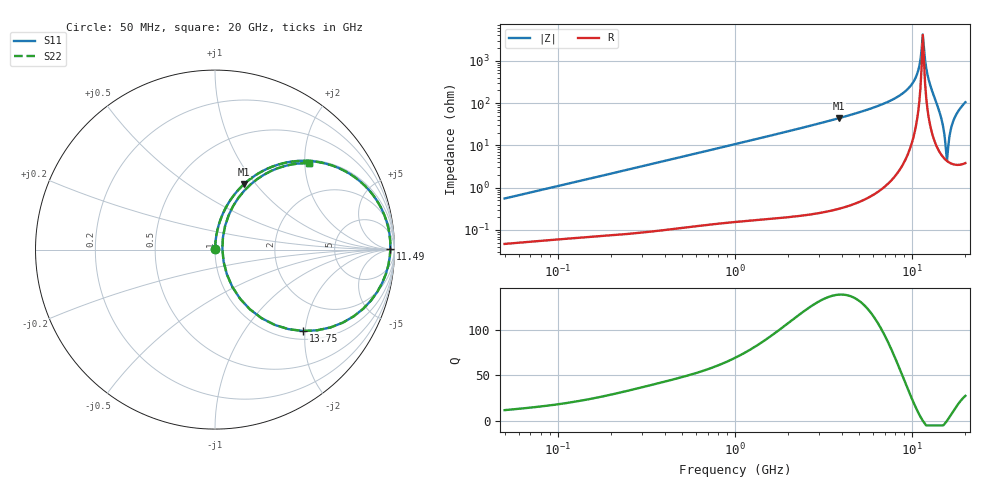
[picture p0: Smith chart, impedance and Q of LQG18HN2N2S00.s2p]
!Murata Part Number: LQG18HN2N2S00
!These Parameters are Measured in Series Mode Connection
!  o--[Z]--o
!Port1  Port2
!  o-------o
!Freq. Start=50[MHz] Stop=20[GHz], 401[Steps]
# Hz S RI R 50
!Freq.(Hz) S11(Real) S11(Imag) S21(Real) S21(Imag) S12(Real) S12(Imag) S22(Real) S22(Imag)
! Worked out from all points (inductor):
!   401 points, 50 MHz to 20 GHz, reference 50 ohm
!   read as one part in series: L = 1.75 nH near 51.52 MHz
!   highest Q = 138 at 3.85 GHz (marker M1), where L = 1.81 nH
!   self-resonance near 11.49 GHz
!   S11 on the Smith chart (normalised r, x): 50 MHz: 1.00, +0.01; 11.49 GHz: 82, +19; 13.75 GHz: 1.19, -1.95; 20 GHz: 1.08, +2.09
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5e7  0.000499 0.00552  0.9995 -0.00552  0.9995 -0.00552  0.000499 0.00552
1.364002e8  0.000878 0.0148  0.9991 -0.0148  0.9991 -0.0148  0.000878 0.0148
3.721004e8  0.00254 0.0397  0.9975 -0.0397  0.9975 -0.0397  0.00254 0.0397
1e9  0.0127 0.1051  0.9873 -0.1051  0.9873 -0.1051  0.0127 0.1051
2.728004e9  0.0837 0.273  0.9163 -0.273  0.9163 -0.273  0.0837 0.273
3.850025e9  0.1621 0.365  0.8379 -0.365  0.8379 -0.365  0.1621 0.365
7.442007e9  0.5504 0.4915  0.4496 -0.4915  0.4496 -0.4915  0.5504 0.4915
1.004137e10  0.8842 0.299  0.1158 -0.299  0.1158 -0.299  0.8842 0.299
1.066139e10  0.9434 0.1927  0.0566 -0.1927  0.0566 -0.1927  0.9434 0.1927
1.131968e10  0.9763 0.0478  0.0237 -0.0478  0.0237 -0.0478  0.9763 0.0478
1.149051e10  0.9772 0.00519  0.0228 -0.00519  0.0228 -0.00519  0.9772 0.00519
1.183995e10  0.9658 -0.0869  0.0342 0.0869  0.0342 0.0869  0.9658 -0.0869
1.220001e10  0.9318 -0.1855  0.0682 0.1855  0.0682 0.1855  0.9318 -0.1855
1.257102e10  0.8689 -0.2841  0.1311 0.2841  0.1311 0.2841  0.8689 -0.2841
1.375312e10  0.4901 -0.4533  0.5099 0.4533  0.5099 0.4533  0.4901 -0.4533
1.460232e10  0.1947 -0.333  0.8053 0.333  0.8053 0.333  0.1947 -0.333
1.527346e10  0.0664 -0.1387  0.9336 0.1387  0.9336 0.1387  0.0664 -0.1387
1.573793e10  0.0411 0.00265  0.9589 -0.00265  0.9589 -0.00265  0.0411 0.00265
1.597544e10  0.0444 0.0699  0.9556 -0.0699  0.9556 -0.0699  0.0444 0.0699
1.670968e10  0.1009 0.2425  0.8991 -0.2425  0.8991 -0.2425  0.1009 0.2425
1.747767e10  0.1984 0.3633  0.8016 -0.3633  0.8016 -0.3633  0.1984 0.3633
2e10  0.5221 0.4816  0.4779 -0.4816  0.4779 -0.4816  0.5221 0.4816
